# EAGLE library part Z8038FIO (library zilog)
Z80 FAMILY DEVICE
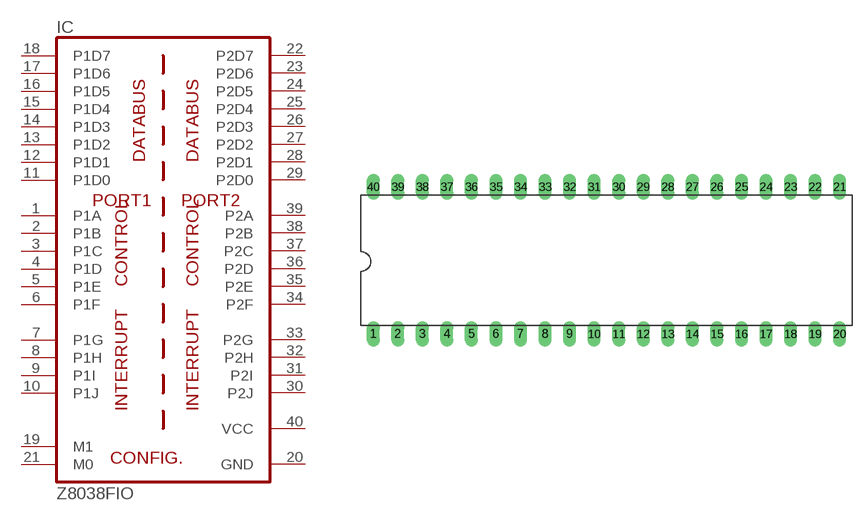
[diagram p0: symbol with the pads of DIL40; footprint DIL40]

Designator prefix IC

## Z8038FIO  [DIL40]
1  P1A  out
2  P1B  in
3  P1C  in
4  P1D  in
5  P1E  in
6  P1F  in
7  P1G  in
8  P1H  out
9  P1I  in
10  P1J  out
11  P1D0
12  P1D1
13  P1D2
14  P1D3
15  P1D4
16  P1D5
17  P1D6
18  P1D7
19  M1  in
20  GND  pwr
21  M0  in
22  P2D7
23  P2D6
24  P2D5
25  P2D4
26  P2D3
27  P2D2
28  P2D1
29  P2D0
30  P2J  out
31  P2I  in
32  P2H  out
33  P2G  in
34  P2F  in
35  P2E  in
36  P2D  in
37  P2C  in
38  P2B  in
39  P2A  out
40  VCC  pwr

## Footprint DIL40 (pad centres in mm)
Dual In Line Package
drill 0.813 long: 1 -24.13,-7.62; 2 -21.59,-7.62; 3 -19.05,-7.62; 4 -16.51,-7.62; 5 -13.97,-7.62; 6 -11.43,-7.62; 7 -8.89,-7.62; 8 -6.35,-7.62; 9 -3.81,-7.62; 10 -1.27,-7.62; 11 1.27,-7.62; 12 3.81,-7.62; 13 6.35,-7.62; 14 8.89,-7.62; 15 11.43,-7.62; 16 13.97,-7.62; 17 16.51,-7.62; 18 19.05,-7.62; 19 21.59,-7.62; 20 24.13,-7.62; 21 24.13,7.62; 22 21.59,7.62; 23 19.05,7.62; 24 16.51,7.62; 25 13.97,7.62; 26 11.43,7.62; 27 8.89,7.62; 28 6.35,7.62; 29 3.81,7.62; 30 1.27,7.62; 31 -1.27,7.62; 32 -3.81,7.62; 33 -6.35,7.62; 34 -8.89,7.62; 35 -11.43,7.62; 36 -13.97,7.62; 37 -16.51,7.62; 38 -19.05,7.62; 39 -21.59,7.62; 40 -24.13,7.62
